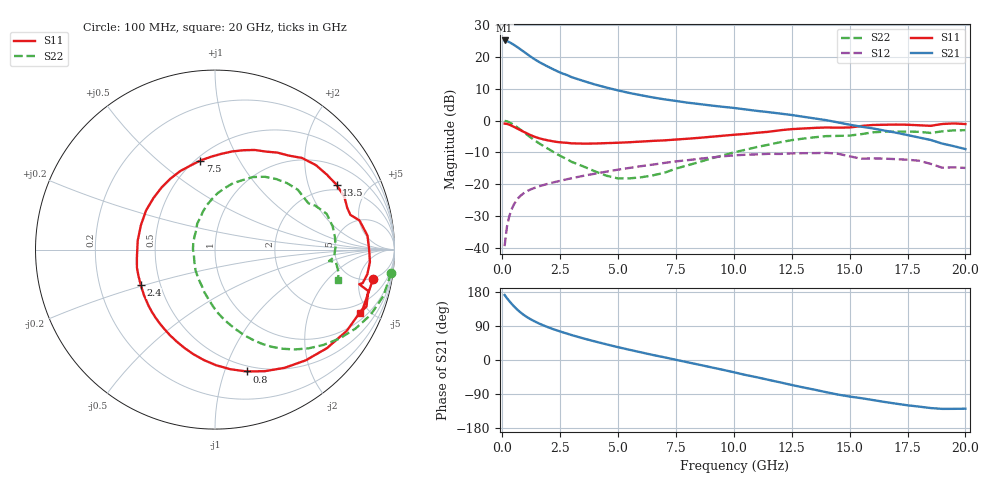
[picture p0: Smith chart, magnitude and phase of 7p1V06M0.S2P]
! Infineon Technologies  Discrete & RF Semiconductors
! bfp620
! VCE =  1.0 V,  IC =  6.0 mA
! Common Emitter S-Parameters:  Sep 2002
# GHz  S  MA  R  50
!  f  S11  S21  S12  S22
! GHz  MAG  ANG  MAG  ANG  MAG  ANG  MAG  ANG
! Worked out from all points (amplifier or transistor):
!   59 points, 100 MHz to 20 GHz, reference 50 ohm
!   highest |S21| = 25.2 dB at 100 MHz (marker M1)
!   |S21| within 3 dB of that: start of sweep to 825 MHz
!   unconditionally stable (mu >= 1): 4.693 GHz to 11.18 GHz; 17 GHz to end of sweep
!   at 1 GHz: K = 0.36, MSG = 21.9 dB, |S12| = -22.5 dB
!   at 5.5 GHz: K = 1.04, MAG = 10.5 dB, |S12| = -14.9 dB
!   at 20 GHz: K = 1.49, MAG = -1.1 dB, |S12| = -14.9 dB
!   S11 on the Smith chart (normalised r, x): 100 MHz: 4.83, -8.01; 800 MHz: 0.45, -1.19; 2.4 GHz: 0.39, -0.19; 7.5 GHz: 0.53, +0.70; 13.5 GHz: 1.75, +3.08; 20 GHz: 1.39, -4.39
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0.1  0.8962 -10.5  18.3 171.5  0.0105 83.2  0.9902 -7.5
0.2  0.8869 -21.5  17.88 163.3  0.0212 79.1  0.9734 -15.4
0.3  0.8624 -31.7  17.22 155.7  0.0309 73.7  0.9403 -22.7
0.4  0.8309 -41.4  16.44 148.6  0.0398 68.7  0.8983 -29.3
0.5  0.7975 -50.7  15.61 141.9  0.0476 64.2  0.8521 -35.6
0.6  0.7643 -59.5  14.78 135.8  0.0546 60.2  0.8046 -41.3
0.8  0.7016 -75.4  13.15 124.9  0.066 53.5  0.7117 -51.4
1  0.6446 -89.4  11.65 115.9  0.0747 48.2  0.6264 -59.8
1.1  0.6187 -95.7  10.97 112.0  0.0783 46.1  0.5876 -63.4
1.4  0.5551 -112.6  9.231 101.8  0.0872 41.1  0.4881 -72.5
1.6  0.5252 -122.4  8.342 96.0  0.0923 38.8  0.4358 -77.7
1.9  0.4938 -135.5  7.3 88.3  0.0994 36.1  0.3734 -84.8
2.4  0.4583 -154.5  5.928 77.3  0.1103 32.5  0.2917 -95.4
3  0.4379 -173.7  4.826 65.7  0.1235 28.7  0.2233 -107.9
3.5  0.4336 173.4  4.216 57.0  0.1348 25.7  0.1896 -118.6
5  0.4473 140.2  2.987 33.8  0.1686 15.8  0.1225 -163.5
7  0.4878 106.2  2.162 7.1  0.2149 0.7  0.1504 134.2
7.5  0.5028 99.4  2.038 0.5  0.2276 -3.8  0.1754 124.4
10.5  0.616 62.4  1.5 -39.4  0.2895 -34.2  0.3468 81.0
13.5  0.7674 28.1  1.079 -78.5  0.3073 -66.0  0.5463 42.7
17  0.8658 -4.6  0.645 -115.2  0.2468 -96.5  0.6722 5.7
20  0.882 -23.5  0.356 -128.5  0.1794 -109.9  0.7056 -13.9
